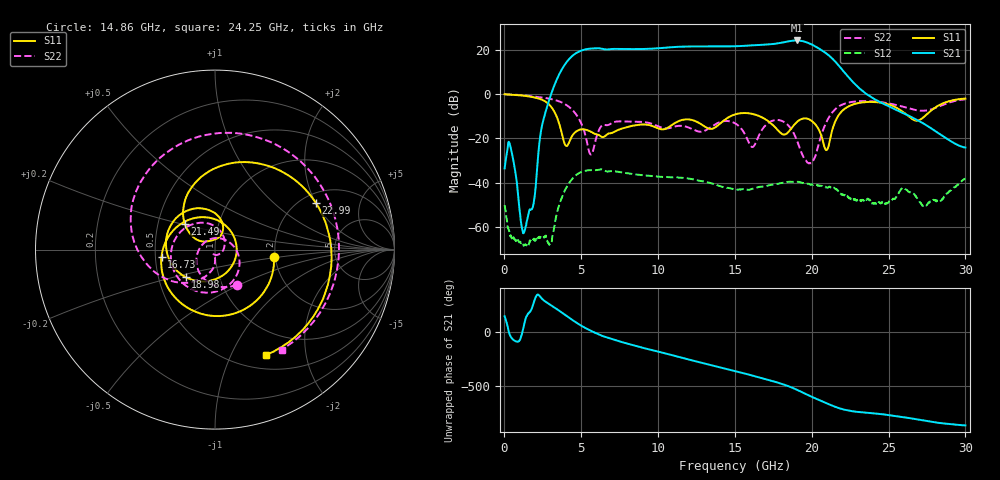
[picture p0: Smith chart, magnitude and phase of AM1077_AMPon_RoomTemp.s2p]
#	Hz	S	DB	R	50
!freq	dBS11	angS11	dBS21	angS21	dBS12	angS12	dBS22	angS22
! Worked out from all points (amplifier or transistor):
!   1601 points, 10 MHz to 30 GHz, reference 50 ohm
!   highest |S21| = 24.2 dB at 19.02 GHz (marker M1)
!   |S21| within 3 dB of that: 10.97 GHz to 20.31 GHz (9.34 GHz wide, 59.7 % of centre)
!   unconditionally stable (mu >= 1): start of sweep to end of sweep
!   at 4.996 GHz: K = 2.87, MAG = 20.0 dB, |S12| = -35.2 dB
!   at 15.01 GHz: K = 5.14, MAG = 22.3 dB, |S12| = -43.1 dB
!   at 30 GHz: K = 108.15, MAG = -16.3 dB, |S12| = -38.3 dB
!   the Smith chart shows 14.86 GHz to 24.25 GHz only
!   S11 on the Smith chart (normalised r, x): 14.86 GHz: 1.97, -0.18; 16.73 GHz: 0.54, -0.05; 18.98 GHz: 0.69, -0.22; 21.49 GHz: 0.69, +0.21; 22.99 GHz: 2.39, +2.01; 24.25 GHz: 0.67, -1.38
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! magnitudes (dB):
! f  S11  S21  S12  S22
! 10 MHz  -0.1  -33.6  -50.2  -0.2
! 403.6 MHz  -0.3  -24.2  -63.8  -0.3
! 1.303 GHz  -0.8  -62.1  -68.2  -0.7
! 1.884 GHz  -1.5  -49.9  -65.6  -1.1
! 2.897 GHz  -4.7  -3.0  -67.9  -2.1
! 4.002 GHz  -23.4  14.0  -42.6  -4.8
! 5.015 GHz  -16.0  19.6  -35.2  -13.5
! 5.633 GHz  -17.1  20.5  -34.4  -27.3
! 6.42 GHz  -19.4  20.3  -34.2  -14.0
! 10.02 GHz  -15.6  20.7  -37.3  -14.6
! 14.86 GHz  -9.6  21.5  -42.8  -12.7
! 15.01 GHz  -9.2  21.6  -43.1  -13.2
! 16.73 GHz  -10.4  22.2  -41.8  -16.6
! 18.98 GHz  -13.0  24.2  -39.7  -20.0
! 19.02 GHz  -12.7  24.2  -39.7  -20.6
! 20.01 GHz  -12.2  22.3  -40.9  -31.1
! 20.95 GHz  -25.3  18.3  -42.2  -12.8
! 21.49 GHz  -13.0  14.9  -42.6  -7.2
! 22.99 GHz  -4.2  3.3  -47.9  -3.3
! 24.25 GHz  -3.7  -3.0  -49.5  -3.5
! 25.01 GHz  -4.7  -5.6  -48.8  -4.3
! 30 GHz  -2.1  -24.2  -38.3  -2.4
